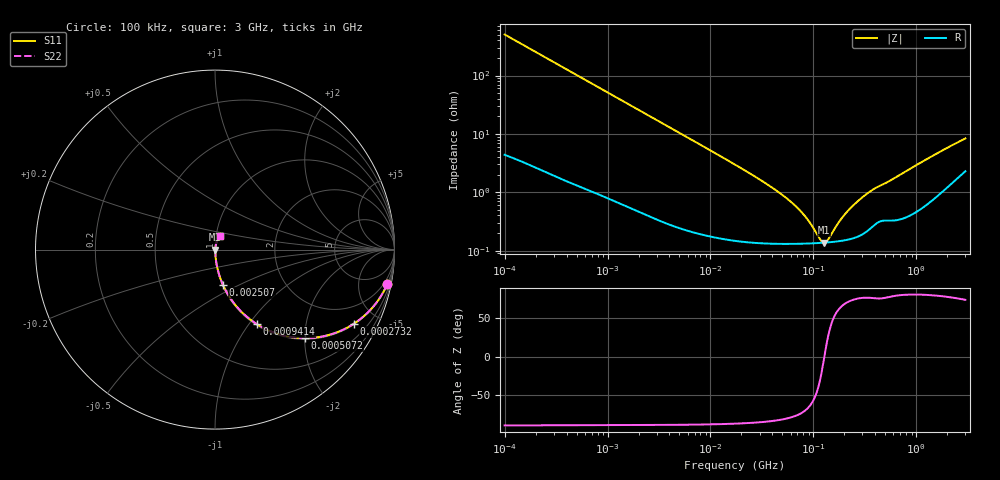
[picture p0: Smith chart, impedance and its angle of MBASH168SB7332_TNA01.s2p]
! MBASH168SB7332_TNA01  S-PARAMETER MODEL  ( Standard Model )
! Model Generated by TAIYO YUDEN Corporation (http://www.ty-top.com)
! Version 1.0
! TAIYO YUDEN Control No. 220601
! Copyright(c) 2013 TAIYO YUDEN CO.,LTD. All Rights Reserved.
! Product Description (link to TY-COMPAS)
! https://ds.yuden.co.jp/TYCOMPAS/or/detail?pn=MBASH168SB7332KTNA01&u=M
! Products Name : Multilayer Ceramic Capacitors
! Characteristics :
!  Capacitance : 3300 [pF] , Rated Voltage : 100 [V] , TCC : X7R
!  Case Size : 1.6 x 0.8 / 0.063 x 0.031 [mm/inch] , Thickness : 0.8 / 0.031 [mm/inch]
!  (Conditions: Temperature = 25 [degC] , DC Bias Voltage = 0 [V])
! External Node Assignments :
!  1  o---| |---o  2
! GND o---------o GND
! Frequency Range : 100kHz  -  3GHz  [ 401 STEP ]
# MHZ S RI R 50
! Freq[MHz].  S11 Real  S11 Imag  S21 Real  S21 Imag  S12 Real  S12 Imag  S22 Real  S22 Imag
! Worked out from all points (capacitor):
!   401 points, 100 kHz to 3 GHz, reference 50 ohm
!   read as one part in series: C = 3.15 nF near 105.3 kHz
!   lowest |Z| = 137 mohm at 126 MHz (marker M1)
!   series resonance near 127.9 MHz, so ESL is about 490 pH
!   S11 on the Smith chart (normalised r, x): 100 kHz: 1, -10; 273.2 kHz: 1.04, -3.72; 507.2 kHz: 1.03, -2.01; 941.4 kHz: 1.02, -1.09; 2.507 MHz: 1.01, -0.41; 3 GHz: 1.05, +0.16
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0.1  0.9607 -0.1901  0.0393 0.1901  0.0393 0.1901  0.9607 -0.1901
0.17181  0.8943 -0.3025  0.1057 0.3025  0.1057 0.3025  0.8943 -0.3025
0.273224  0.773 -0.4134  0.227 0.4134  0.227 0.4134  0.773 -0.4134
0.507162  0.5027 -0.4936  0.4973 0.4936  0.4973 0.4936  0.5027 -0.4936
0.562235  0.4524 -0.4911  0.5476 0.4911  0.5476 0.4911  0.4524 -0.4911
0.941399  0.2321 -0.4147  0.7679 0.4147  0.7679 0.4147  0.2321 -0.4147
1.458987  0.1148 -0.3105  0.8852 0.3105  0.8852 0.3105  0.1148 -0.3105
2.506689  0.0443 -0.1965  0.9557 0.1965  0.9557 0.1965  0.0443 -0.1965
3.161081  0.0292 -0.1586  0.9708 0.1586  0.9708 0.1586  0.0292 -0.1586
6.674626  0.00807 -0.0772  0.9919 0.0772  0.9919 0.0772  0.00807 -0.0772
17.7727  0.00229 -0.0289  0.9977 0.0289  0.9977 0.0289  0.00229 -0.0289
55.23785  0.00136 -0.00772  0.9986 0.00772  0.9986 0.00772  0.00136 -0.00772
75.25761  0.00133 -0.00455  0.9987 0.00455  0.9987 0.00455  0.00133 -0.00455
97.38194  0.00134 -0.00226  0.9987 0.00226  0.9987 0.00226  0.00134 -0.00226
116.6348  0.00135 -0.000755  0.9986 0.000755  0.9986 0.000755  0.00135 -0.000755
126.0104  0.00137 -0.00012  0.9986 0.00012  0.9986 0.00012  0.00137 -0.00012
139.694  0.00139 0.000725  0.9986 -0.000725  0.9986 -0.000725  0.00139 0.000725
185.4806  0.00147 0.00313  0.9985 -0.00313  0.9985 -0.00313  0.00147 0.00313
252.704  0.00169 0.00608  0.9983 -0.00608  0.9983 -0.00608  0.00169 0.00608
362.5028  0.00254 0.0102  0.9975 -0.0102  0.9975 -0.0102  0.00254 0.0102
547.5153  0.00348 0.0151  0.9965 -0.0151  0.9965 -0.0151  0.00348 0.0151
3000  0.0284 0.0763  0.9716 -0.0763  0.9716 -0.0763  0.0284 0.0763
